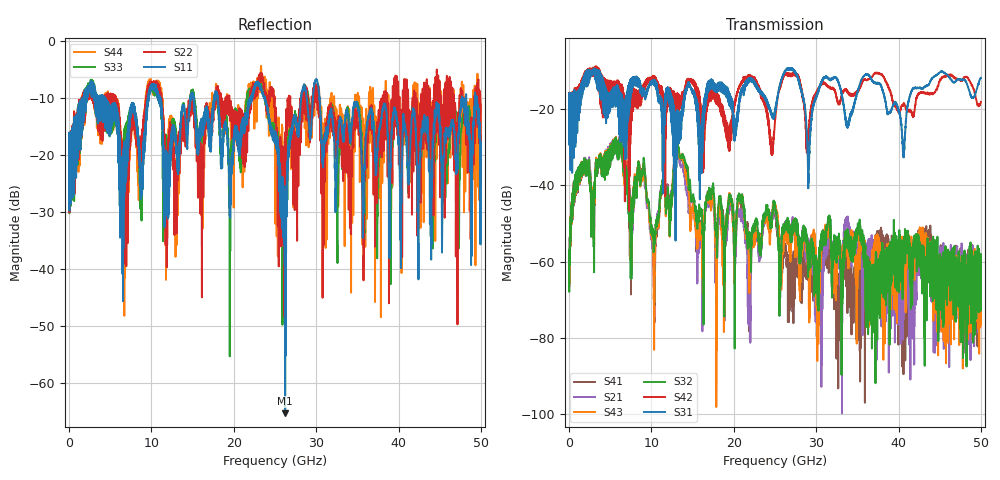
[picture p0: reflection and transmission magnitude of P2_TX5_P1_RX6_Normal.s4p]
!Keysight Technologies,N5225B,MY57041031,A.13.20.10
!Date: Friday, May 31, 2019 11:23:33
!Correction: S11(Full 4 Port(1,2,3,4))
!S12(Full 4 Port(1,2,3,4))
!S13(Full 4 Port(1,2,3,4))
!S14(Full 4 Port(1,2,3,4))
!S21(Full 4 Port(1,2,3,4))
!S22(Full 4 Port(1,2,3,4))
!S23(Full 4 Port(1,2,3,4))
!S24(Full 4 Port(1,2,3,4))
!S31(Full 4 Port(1,2,3,4))
!S32(Full 4 Port(1,2,3,4))
!S33(Full 4 Port(1,2,3,4))
!S34(Full 4 Port(1,2,3,4))
!S41(Full 4 Port(1,2,3,4))
!S42(Full 4 Port(1,2,3,4))
!S43(Full 4 Port(1,2,3,4))
!S44(Full 4 Port(1,2,3,4))
!S4P File: Measurements: <S11,S12,S13,S14>,
!<S21,S22,S23,S24>,
!<S31,S32,S33,S34>,
!<S41,S42,S43,S44>:
# Hz S  dB  R 50.0
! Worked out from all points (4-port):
!   5000 points, 10 MHz to 50 GHz, reference 50 ohm
!   strongest paths, dB at 10 MHz, 12.51 GHz, 25.01 GHz, 37.51 GHz, 50 GHz:
!     S31: -19.5, -17.7, -20.9, -13.2, -11.7
!     S42: -19.4, -15.5, -22.8, -10.6, -18.1
!     S32: -61.5, -43.0, -45.6, -65.1, -72.6
!     S43: -59.2, -41.9, -45.7, -54.8, -65.7
!     S21: -56.9, -41.5, -46.7, -64.3, -58.1
!     S41: -65.0, -44.0, -47.6, -54.8, -63.9
!   lowest |S11| = -65.3 dB at 26.24 GHz (marker M1), VSWR 1.00, Z = 49.9 + j0.00555 ohm
!   |S11| at or under -10 dB: 4.282 GHz to 9.568 GHz (5.285 GHz wide, 76.3 % of centre); 23.74 GHz to 28.18 GHz (4.439 GHz wide, 17.1 % of centre); 30.41 GHz to 47.7 GHz (17.29 GHz wide, 44.3 % of centre)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
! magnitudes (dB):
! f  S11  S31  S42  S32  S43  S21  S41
! 10 MHz  -19.8  -19.5  -19.4  -61.5  -59.2  -56.9  -65.0
! 5.55 GHz  -11.7  -18.3  -13.7  -28.6  -28.4  -28.5  -28.9
! 10.25 GHz  -8.0  -12.8  -12.0  -53.1  -62.6  -59.9  -56.4
! 13.11 GHz  -19.6  -20.8  -15.8  -29.6  -29.7  -30.3  -30.3
! 21.85 GHz  -10.6  -12.7  -11.6  -55.6  -62.5  -75.3  -66.5
! 26.24 GHz  -65.3  -9.9  -10.5  -51.2  -52.6  -51.1  -57.3
! 50 GHz  -19.3  -11.7  -18.1  -72.6  -65.7  -58.1  -63.9
